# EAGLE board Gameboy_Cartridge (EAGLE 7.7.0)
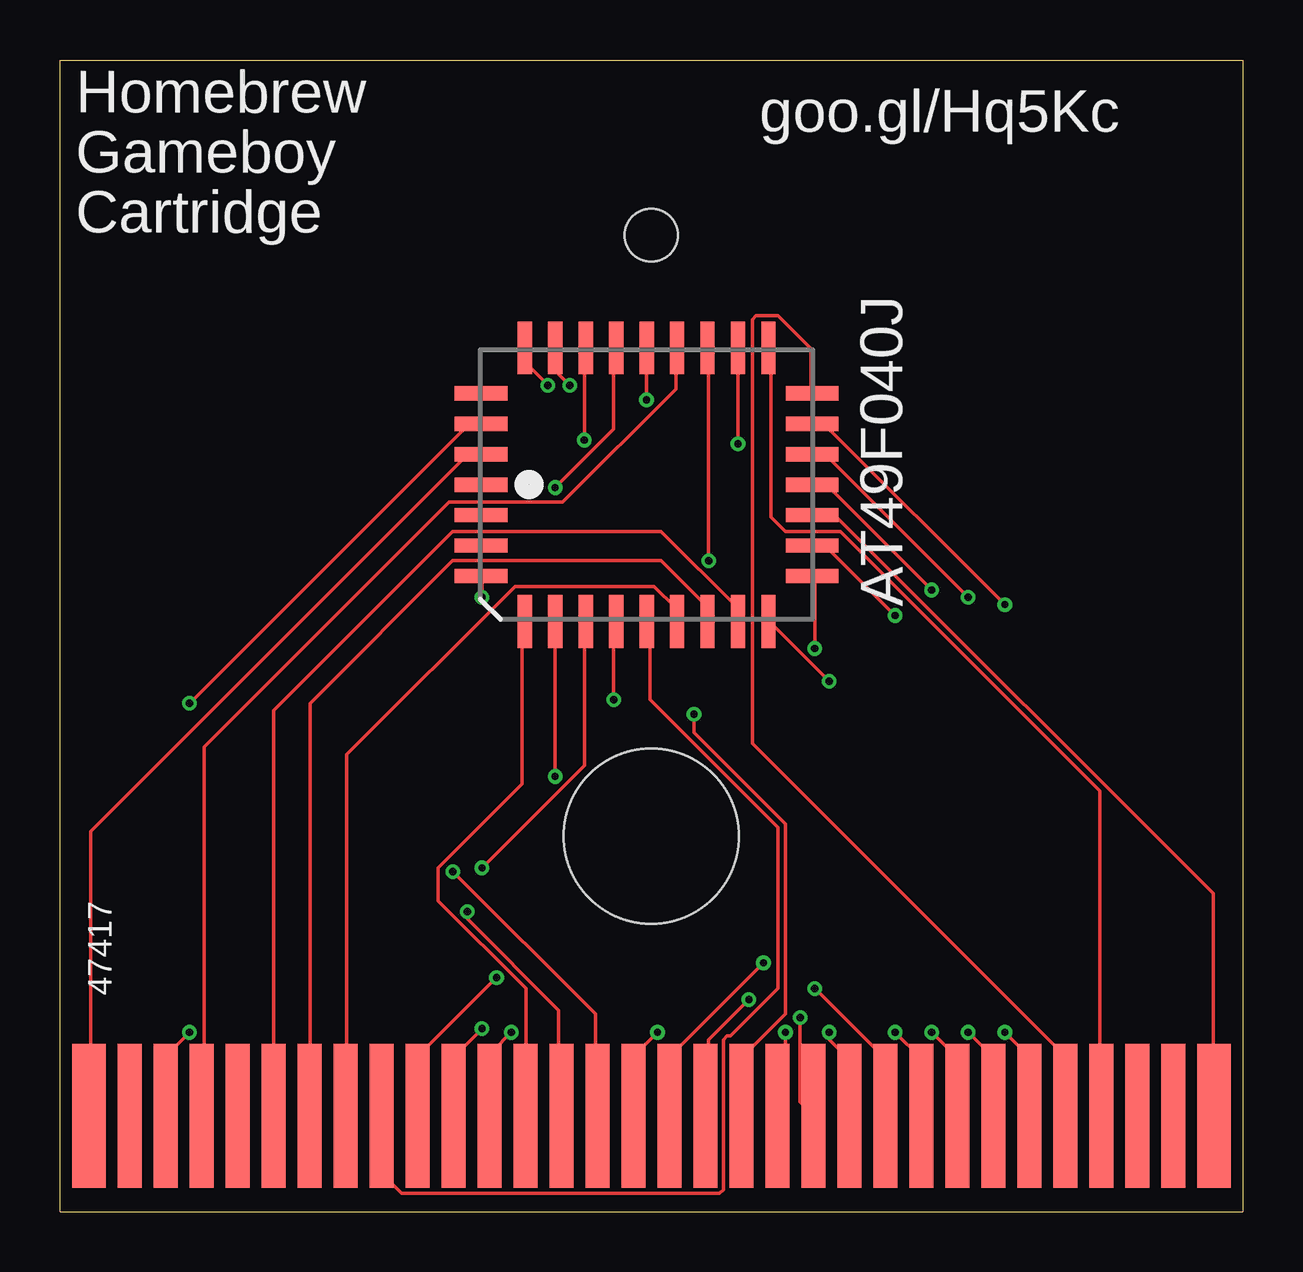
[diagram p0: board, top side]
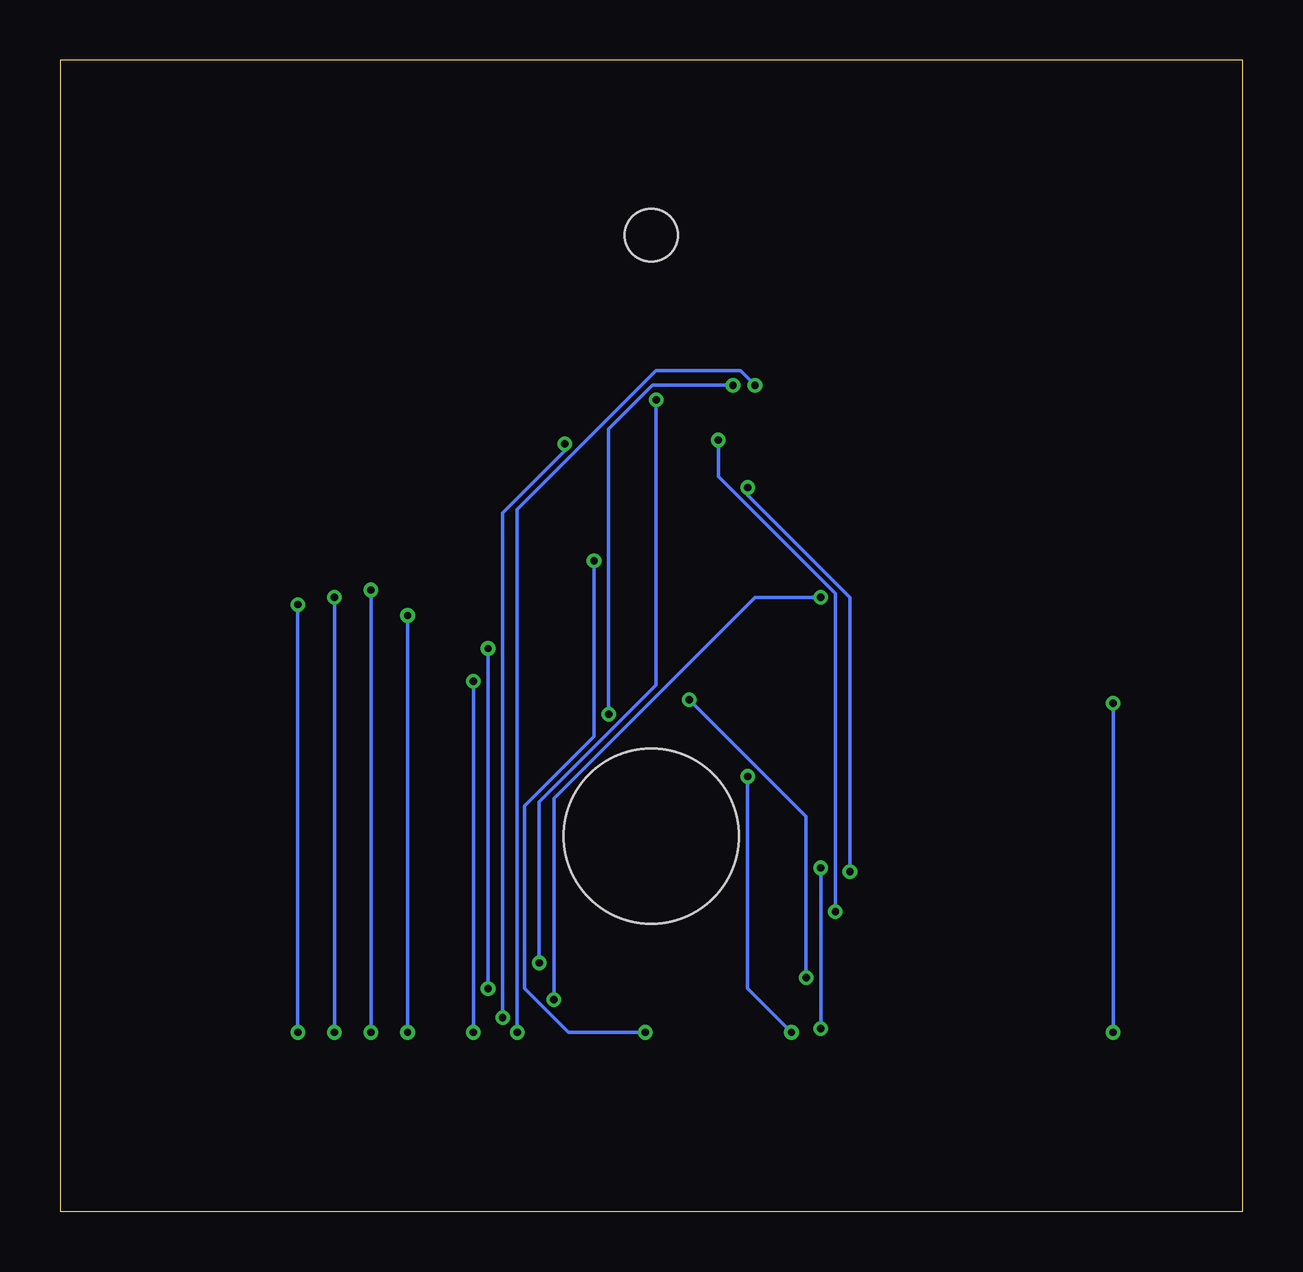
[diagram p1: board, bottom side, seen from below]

Size 49.3 x 48 mm. Coordinates in mm from the lower left corner, seen from the top.
Outline: 49.3,48 49.3,0 0,0 0,48 49.3,48
Copper layers (1*16): Top 0.035mm / dielectric 1.5mm / Bottom 0.035mm
Design rules "default": minimum track width 6mil, minimum drill 12mil, track to track 6mil, track to pad 6mil, pad to pad 6mil, via to via 6mil, smd to smd 0mil, copper to edge 10mil, drill to drill 10mil, minimum pad ring 10mil, minimum via ring 6mil, stop-mask expansion 2mil, vias tented up to drill 100mil, thermal gap 10mil
Holes 7.3 mm at 24.65,15.65
Holes 2.2 mm at 24.65,40.7

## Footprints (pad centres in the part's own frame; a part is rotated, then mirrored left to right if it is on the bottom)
PLCC32R = smd 0.6 x 2.2: 1 0,6.9; 2 -1.27,6.9; 3 -2.54,6.9; 4 -3.81,6.9; 14 -3.81,-6.9; 15 -2.54,-6.9; 16 -1.27,-6.9; 17 0,-6.9; 18 1.27,-6.9; 19 2.54,-6.9; 20 3.81,-6.9; 30 3.81,6.9; 31 2.54,6.9; 32 1.27,6.9 | smd 2.2 x 0.6: 5 -5.7,5.08; 6 -5.7,3.81; 7 -5.7,2.54; 8 -5.7,1.27; 9 -5.7,0; 10 -5.7,-1.27; 11 -5.7,-2.54; 12 -5.7,-3.81; 13 -5.7,-5.08; 21 5.7,-5.08; 22 5.7,-3.81; 23 5.7,-2.54; 24 5.7,-1.27; 25 5.7,0; 26 5.7,1.27; 27 5.7,2.54; 28 5.7,3.81; 29 5.7,5.08
CONNECTOR = smd 1.4 x 6: 1 0.7,-3; 32 47.6,-3 | smd 1 x 6: 2 2.4,-3; 3 3.9,-3; 4 5.4,-3; 5 6.9,-3; 6 8.4,-3; 7 9.9,-3; 8 11.4,-3; 9 12.9,-3; 10 14.4,-3; 11 15.9,-3; 12 17.4,-3; 13 18.9,-3; 14 20.4,-3; 15 21.9,-3; 16 23.4,-3; 17 24.9,-3; 18 26.4,-3; 19 27.9,-3; 20 29.4,-3; 21 30.9,-3; 22 32.4,-3; 23 33.9,-3; 24 35.4,-3; 25 36.9,-3; 26 38.4,-3; 27 39.9,-3; 28 41.4,-3; 29 42.9,-3; 30 44.4,-3; 31 45.9,-3

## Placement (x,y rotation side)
IC1  AT49F040J  [PLCC32R]  24.45,30.3 90 top
U$1  CONNECTOR  [CONNECTOR]  0.5,7 0 top

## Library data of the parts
IC1 U$1 = gameboy

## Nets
3: IC1.31 U$1.3
4: IC1.24 U$1.4
5: U$1.5
6: IC1.12 U$1.6
7: IC1.11 U$1.7
8: IC1.10 U$1.8
9: IC1.9 U$1.9
10: IC1.8 U$1.10
11: IC1.7 U$1.11
12: IC1.6 U$1.12
13: IC1.5 U$1.13
14: IC1.27 U$1.14
15: IC1.26 U$1.15
16: IC1.23 U$1.16
17: IC1.25 U$1.17
18: IC1.4 U$1.18
19: IC1.28 U$1.19
20: IC1.29 U$1.20
21: IC1.22 U$1.21
22: IC1.13 U$1.22
23: IC1.14 U$1.23
24: IC1.15 U$1.24
25: IC1.17 U$1.25
26: IC1.18 U$1.26
27: IC1.19 U$1.27
28: IC1.20 U$1.28
29: IC1.21 U$1.29
30: U$1.30
31: U$1.31
GND: IC1.16 U$1.32
VDD: IC1.32 U$1.1

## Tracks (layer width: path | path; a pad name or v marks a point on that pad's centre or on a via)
3  (via drill 0.3)
  Top 0.152: v5.4,21.18 16.98,32.77 17.44,32.77 IC1.31 | v5.4,7.47 4.48,6.55 4.48,4.12 U$1.3
  Bottom 0.152: v5.4,7.47 v5.4,21.18
4
  Top 0.152: IC1.24 25.67,35.97 25.67,34.29 20.94,29.57 16.22,29.57 6.01,19.36 6.01,4.12 U$1.4
6
  Top 0.152: IC1.12 28.26,24.69 28.26,25.15 25.06,28.35 16.37,28.35 8.9,20.88 8.9,4.12 U$1.6
7
  Top 0.152: IC1.11 26.89,24.69 26.89,25.3 25.06,27.13 16.37,27.13 10.43,21.18 10.43,4.12 U$1.7
8
  Top 0.152: IC1.10 25.67,24.69 25.67,25.15 24.75,26.06 18.96,26.06 11.95,19.05 11.95,4.12 U$1.8
9
  Top 0.152: IC1.9 24.6,24.54 24.6,21.34 29.93,16 29.93,9.3 27.95,7.32 27.8,7.32 27.65,7.16 27.65,0.91 27.5,0.76 14.24,0.76 13.48,1.52 13.48,3.96 U$1.9
10  (via drill 0.3)
  Top 0.152: v23.08,21.34 23.08,24.54 IC1.8 | v18.2,9.75 15,6.55 15,4.12 U$1.10
  Bottom 0.152: v23.08,21.34 18.2,16.46 v18.2,9.75
11  (via drill 0.3)
  Top 0.152: v17.59,14.33 21.86,18.59 21.86,24.54 IC1.7 | v17.59,7.62 16.52,6.55 16.52,4.12 U$1.11
  Bottom 0.152: v17.59,7.62 v17.59,14.33
12  (via drill 0.3)
  Top 0.152: v20.64,18.14 20.64,24.54 IC1.6 | v18.81,7.47 18.05,6.71 18.05,4.12 U$1.12
  Bottom 0.152: v20.64,18.14 20.64,9.3 v18.81,7.47
13
  Top 0.152: IC1.5 19.27,24.54 19.27,17.83 15.76,14.33 15.76,12.95 19.42,9.3 19.42,4.12 U$1.13
14  (via drill 0.3)
  Top 0.152: v21.86,32.16 21.86,35.97 IC1.27 | v16.98,12.5 16.98,12.19 20.79,8.38 20.79,4.12 U$1.14
  Bottom 0.152: v21.86,32.16 21.86,30.63 16.98,25.76 v16.98,12.5
15  (via drill 0.3)
  Top 0.152: v20.64,30.18 23.08,32.61 23.08,35.97 IC1.26 | v16.37,14.17 22.31,8.23 22.31,4.12 U$1.15
  Bottom 0.152: v20.64,30.18 20.64,29.87 16.37,25.6 v16.37,14.17
16  (via drill 0.3)
  Top 0.152: v27.04,27.13 27.04,35.97 IC1.23 | v24.91,7.47 23.99,6.55 23.99,4.12 U$1.16
  Bottom 0.152: v27.04,27.13 27.04,19.81 29.93,16.92 29.93,9.3 28.11,7.47 v24.91,7.47
17  (via drill 0.3)
  Top 0.152: v24.45,33.83 24.45,35.97 IC1.25 | v29.32,10.36 25.51,6.55 25.51,4.12 U$1.17
  Bottom 0.152: v24.45,33.83 24.45,21.95 29.32,17.07 v29.32,10.36
18  (via drill 0.3)
  Top 0.152: v17.59,25.6 17.59,26.36 IC1.4 | v28.72,8.84 27.04,7.16 27.04,4.12 U$1.18
  Bottom 0.152: v17.59,25.6 20.33,25.6 28.72,17.22 v28.72,8.84
19  (via drill 0.3)
  Top 0.152: v21.25,34.44 20.79,34.9 20.79,35.97 IC1.28 | v26.43,20.73 26.43,19.96 30.24,16.15 30.24,8.23 28.41,6.4 28.41,4.12 U$1.19
  Bottom 0.152: v21.25,34.44 24.6,34.44 26.43,32.61 v26.43,20.73
20  (via drill 0.3)
  Top 0.152: v20.33,34.44 19.42,35.36 19.42,35.97 IC1.29 | v30.24,7.47 30.24,4.42 29.93,4.12 U$1.20
  Bottom 0.152: v20.33,34.44 20.94,35.05 24.45,35.05 30.24,29.26 v30.24,7.47
21  (via drill 0.3)
  Top 0.152: v28.26,32 28.26,35.97 IC1.22 | v30.85,8.08 30.85,4.57 31.31,4.12 U$1.21
  Bottom 0.152: v28.26,32 28.26,31.7 30.85,29.11 v30.85,8.08
22  (via drill 0.3)
  Top 0.152: v32.07,22.1 29.63,24.54 IC1.13 | v32.07,7.47 32.07,7.16 32.83,6.4 32.83,4.12 U$1.22
  Bottom 0.152: v32.07,7.47 v32.07,22.1
23  (via drill 0.3)
  Top 0.152: v31.46,23.47 31.46,26.36 IC1.14 | v31.46,9.3 34.35,6.4 34.35,4.12 U$1.23
  Bottom 0.152: v31.46,9.3 v31.46,23.47
24  (via drill 0.3)
  Top 0.152: v34.81,24.84 31.92,27.74 31.46,27.74 IC1.15 | v34.81,7.47 35.88,6.4 35.88,4.12 U$1.24
  Bottom 0.152: v34.81,7.47 v34.81,24.84
25  (via drill 0.3)
  Top 0.152: v36.34,25.91 32.07,30.18 31.46,30.18 IC1.17 | v36.34,7.47 37.25,6.55 37.25,4.12 U$1.25
  Bottom 0.152: v36.34,7.47 v36.34,25.91
26  (via drill 0.3)
  Top 0.152: v37.86,25.6 31.92,31.55 31.46,31.55 IC1.18 | v37.86,7.47 38.77,6.55 38.77,4.12 U$1.26
  Bottom 0.152: v37.86,7.47 v37.86,25.6
27  (via drill 0.3)
  Top 0.152: v39.38,25.3 31.92,32.77 31.46,32.77 IC1.19 | v39.38,7.47 40.3,6.55 40.3,4.12 U$1.27
  Bottom 0.152: v39.38,7.47 v39.38,25.3
28
  Top 0.152: IC1.20 31.31,34.14 31.31,35.97 29.93,37.34 29.02,37.34 28.87,37.19 28.87,19.51 41.82,6.55 41.82,4.12 U$1.28
29
  Top 0.152: IC1.21 29.63,35.97 29.63,28.96 30.24,28.35 32.53,28.35 43.35,17.53 43.35,4.12 U$1.29
GND
  Top 0.152: IC1.16 31.46,28.96 32.37,28.96 48.07,13.26 48.07,4.12 U$1.32
VDD
  Top 0.152: IC1.32 17.44,31.55 16.98,31.55 1.28,15.85 1.28,4.12 U$1.1

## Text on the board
tPlace: Homebrew | goo.gl/Hq5Kc | Gameboy | Cartridge | 47417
